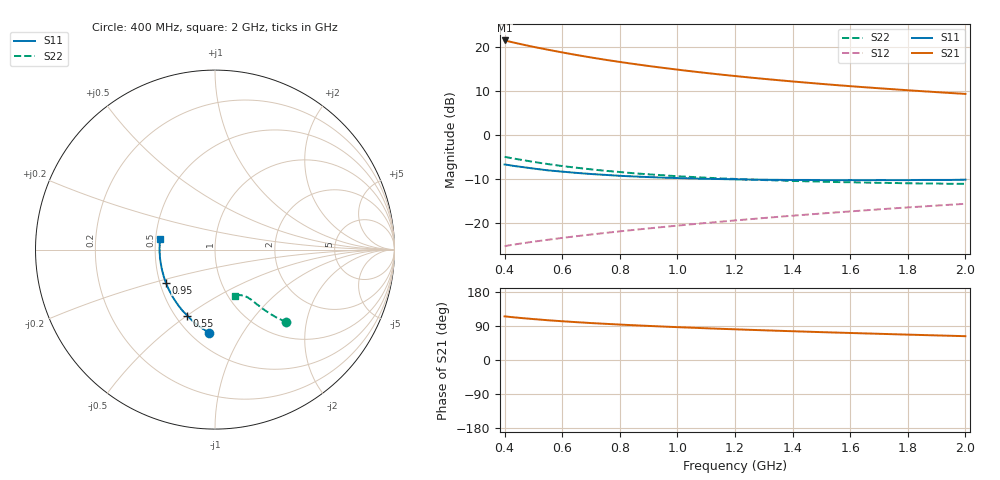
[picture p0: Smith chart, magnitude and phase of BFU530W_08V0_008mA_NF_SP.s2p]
! Filename:  P:\Prog\Test\Noise\ATS_data\Testdata_Net\06 Compressed Noise after Statistics\BFU530W_APM2013_09_A05_08p0V_008mA_NF_CM01_D.sf
! Date/Time: Tue 26/Mar/2013 18:06:03
! BFU530W_APM2013_09_A05_08p0V_1to25mA_NF_CM01_Bias5_R.sf
! Noise Parameter Data File
! BFU530W_APM2013_09_A05_08p0V_1to25mA_NF_CM01
! Date/time: Thu Mar 21 21:44:48 2013
! VAR V_out= 8.000000
! VAR I_out= 7.990000
! VAR V_in= 0.814600
! VAR I_in= 0.080505
! Device data file deembeded for feedlines and parallel
! Original file: \06 Compressed Noise after Statistics\BFU530W_APM2013_09_A05_08p0V_008mA_NF_CM01_R.sf
! Feed-files: PR019V01_070313_Feed1.s2p, PR019V01_070313_Feed2.s2p
! Parallel-file: PR019V01_070313_Par.s2p
# MHz S MA R 50
!  Freq-MHz  S11-mag  S11-arg  S21-mag  S21-arg  S12-mag  S12-arg  S22-mag  S22-arg
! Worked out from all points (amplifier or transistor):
!   37 points, 400 MHz to 2 GHz, reference 50 ohm
!   highest |S21| = 21.4 dB at 400 MHz (marker M1)
!   |S21| within 3 dB of that: start of sweep to 625.2 MHz
!   unconditionally stable (mu >= 1): 1.537 GHz to end of sweep
!   at 500 MHz: K = 0.65, MSG = 22.0 dB, |S12| = -24.1 dB
!   at 1.1 GHz: K = 0.94, MSG = 17.0 dB, |S12| = -19.9 dB
!   at 2 GHz: K = 1.02, MAG = 11.6 dB, |S12| = -15.6 dB
!   lowest NFmin = 0.70 dB at 420 MHz
!   S11 on the Smith chart (normalised r, x): 400 MHz: 0.61, -0.72; 550 MHz: 0.57, -0.50; 950 MHz: 0.54, -0.22; 2 GHz: 0.53, +0.07
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400  0.4643 -93.9  11.72 115.2  0.05533 57.9  0.566 -45.3
420  0.4536 -96.8  11.32 113.6  0.05681 57.7  0.5505 -46.1
440  0.4433 -99.6  10.94 112.1  0.05819 57.5  0.5357 -46.8
480  0.4261 -104.7  10.24 109.3  0.06085 57.4  0.5093 -47.9
500  0.4176 -107.2  9.923 108.0  0.06214 57.3  0.4965 -48.4
550  0.3985 -112.8  9.217 104.9  0.06536 57.4  0.4692 -49.4
600  0.3852 -118.2  8.584 102.2  0.06861 57.6  0.4455 -50.2
650  0.3728 -123.0  8.022 99.8  0.07179 57.8  0.4264 -51.0
700  0.3622 -127.5  7.529 97.5  0.07494 58.1  0.4091 -51.6
750  0.3539 -131.7  7.088 95.5  0.0781 58.5  0.3935 -52.1
800  0.3455 -135.7  6.697 93.5  0.08137 58.9  0.3815 -52.7
850  0.3397 -139.5  6.346 91.7  0.08459 59.2  0.3691 -53.1
950  0.3297 -146.0  5.744 88.3  0.09117 59.9  0.3505 -53.9
1050  0.3227 -152.1  5.244 85.2  0.09782 60.6  0.3353 -54.7
1150  0.3175 -157.7  4.824 82.3  0.1046 61.1  0.3229 -55.6
1200  0.315 -160.1  4.642 81.0  0.1081 61.3  0.3187 -56.1
1250  0.3133 -162.7  4.47 79.7  0.1116 61.5  0.3135 -56.5
1350  0.3109 -167.1  4.168 77.1  0.1188 61.9  0.3063 -57.5
1500  0.3089 -173.4  3.783 73.5  0.1295 62.1  0.297 -59.3
1650  0.3085 -179.2  3.467 70.2  0.1405 62.3  0.2898 -61.0
1750  0.3089 177.4  3.29 68.0  0.148 62.3  0.2867 -62.3
2000  0.3126 169.3  2.916 62.9  0.1668 62.0  0.2803 -66.0
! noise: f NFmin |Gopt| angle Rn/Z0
400  0.7022  0.05867  74.87  0.0909
460  0.7177  0.05002  81.67  0.0906
600  0.7382  0.0602  85.39  0.0926
800  0.7601  0.08736  115  0.0858
1000  0.7972  0.1016  125  0.085
1200  0.8155  0.1391  136.8  0.0807
1400  0.8554  0.1519  144.9  0.0804
1600  0.8795  0.1792  156.5  0.0712
1800  0.8988  0.2075  165.7  0.0699
2000  0.9128  0.2218  173.8  0.0724
